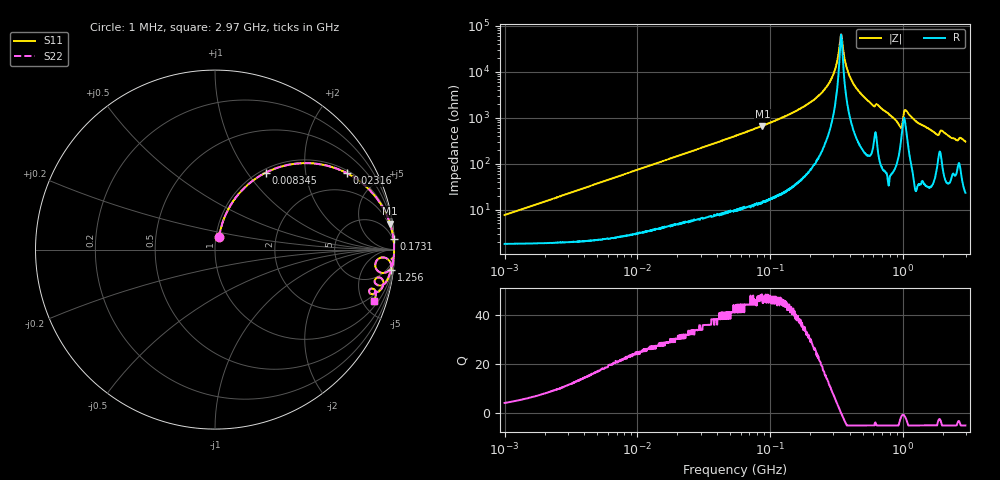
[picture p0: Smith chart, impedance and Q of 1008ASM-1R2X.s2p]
!s-Parameter Generated by FASTRON Sdn. Bhd.
!FASTRON P/N : 1008ASM-1R2X
!Keysight Technologies: E4991B_MY54100416_A.01.15
!Date: Tue Nov 21 09:45:12 2023
!Version  :Rev00  Wed Nov 22 15:04:50 2023
!Data & Calibration Information:
!Freq  S11  S21  S12  S22
!PortZ  Port1:50+j0  Port2:50+j0
!When reading reference impedance value at option line is always used.
! Remarks : This data is being provided solely for informational purposes.
# Hz S dB R 50
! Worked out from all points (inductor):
!   1599 points, 1 MHz to 2.97 GHz, reference 50 ohm
!   read as one part in series: L = 1.19 uH near 1.036 MHz
!   highest Q = 46.9 at 87.67 MHz (marker M1), where L = 1.21 uH
!   self-resonance near 343.7 MHz
!   S11 on the Smith chart (normalised r, x): 1 MHz: 1.04, +0.15; 8.345 MHz: 1.06, +1.23; 23.16 MHz: 1.11, +3.38; 173.1 MHz: 2, +33; 1.256 GHz: 2, -17; 2.97 GHz: 1.47, -6.04
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1000000  -22.50 72.2  -0.18 -4.2  -0.18 -4.2  -22.50 72.2
3804036  -11.50 70.4  -0.50 -15.5  -0.50 -15.5  -11.50 70.4
8345207  -5.77 56.5  -1.57 -31.0  -1.57 -31.0  -5.77 56.5
1.439846e7  -2.93 42.4  -3.41 -45.5  -3.41 -45.5  -2.93 42.4
2.316168e7  -1.42 30.1  -5.98 -58.1  -5.98 -58.1  -1.42 30.1
5.477226e7  -0.31 13.8  -12.40 -74.8  -12.40 -74.8  -0.31 13.8
8.766808e7  -0.12 8.5  -16.60 -80.3  -16.60 -80.3  -0.12 8.5
1.731398e8  -0.03 3.5  -24.40 -84.9  -24.40 -84.9  -0.03 3.5
2.073156e8  -0.02 2.5  -27.30 -85.5  -27.30 -85.5  -0.02 2.5
2.898922e8  -0.01 0.8  -36.90 -83.2  -36.90 -83.2  -0.01 0.8
3.140564e8  -0.01 0.4  -42.30 -78.4  -42.30 -78.4  -0.01 0.4
3.436571e8  -0.01 0.0  -56.30 -1.7  -56.30 -1.7  -0.01 0.0
3.836505e8  -0.01 -0.5  -40.70 79.3  -40.70 79.3  -0.01 -0.5
4.347762e8  -0.02 -1.1  -34.00 83.7  -34.00 83.7  -0.02 -1.1
5.899715e8  -0.06 -3.0  -25.70 81.5  -25.70 81.5  -0.06 -3.0
7.846996e8  -0.05 -4.7  -21.70 83.7  -21.70 83.7  -0.05 -4.7
9.538021e8  -0.51 -7.9  -16.70 63.1  -16.70 63.1  -0.51 -7.9
1.054198e9  -0.28 -3.4  -23.60 60.1  -23.60 60.1  -0.28 -3.4
1.255985e9  -0.09 -6.7  -18.70 81.6  -18.70 81.6  -0.09 -6.7
1.791767e9  -0.49 -12.2  -13.40 69.2  -13.40 69.2  -0.49 -12.2
1.970482e9  -0.47 -10.1  -14.90 67.8  -14.90 67.8  -0.47 -10.1
2.970126e9  -0.65 -17.8  -10.30 67.8  -10.30 67.8  -0.65 -17.8
